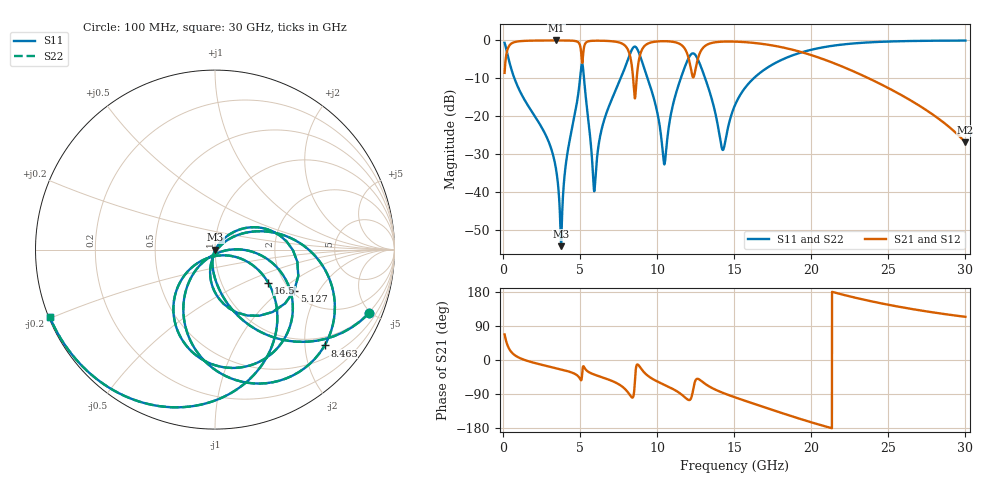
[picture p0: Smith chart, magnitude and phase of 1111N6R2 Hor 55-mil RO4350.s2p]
# GHz S MA R 50
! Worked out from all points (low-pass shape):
!   3201 points, 100 MHz to 30 GHz, reference 50 ohm
!   highest |S21| = -0.02 dB at 3.464 GHz (marker M1); lowest = -26.9 dB at 30 GHz (marker M2)
!   |S21| within 3 dB of the highest: 248.2 MHz to 5.061 GHz (4.813 GHz wide, 181 % of centre); 12.81 GHz to 19.3 GHz (6.488 GHz wide, 40.4 % of centre)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
!   lowest |S11| = -54.3 dB at 3.763 GHz (marker M3), VSWR 1.00, Z = 50.2 - j0.0862 ohm
!   |S11| at or under -10 dB: 733.6 MHz to 4.999 GHz (4.265 GHz wide, 149 % of centre); 5.251 GHz to 7.637 GHz (2.385 GHz wide, 37 % of centre); 13.11 GHz to 16.27 GHz (3.152 GHz wide, 21.5 % of centre)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
!   |S22| runs from -54.3 to 0.0 dB; largest |S21 - S12| = 0
!   S11 on the Smith chart (normalised r, x): 100 MHz: 0.95, -4.84; 5.127 GHz: 2.07, -1.26; 8.463 GHz: 0.78, -2.45; 16.5 GHz: 1.66, -0.69; 30 GHz: 0.00, -0.20
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0.1  0.9278 -22.6  0.3727 67.4  0.3727 67.4  0.9278 -22.6
0.810125  0.2879 -78.6  0.957 11.3  0.957 11.3  0.2879 -78.6
3.46375  0.01843 -107.0  0.9979 -21.8  0.9979 -21.8  0.01843 -107.0
3.76275  0.001918 -26.6  0.9976 -24.8  0.9976 -24.8  0.001918 -26.6
5.089563  0.4641 -8.5  0.6097 -51.8  0.6097 -51.8  0.4641 -8.5
5.126938  0.4971 -27.4  0.5078 -39.4  0.5078 -39.4  0.4971 -27.4
5.939844  0.01075 -15.4  0.9895 -38.8  0.9895 -38.8  0.01075 -15.4
6.500469  0.08074 37.7  0.9881 -46.7  0.9881 -46.7  0.08074 37.7
7.817938  0.391 11.8  0.8846 -73.0  0.8846 -73.0  0.391 11.8
8.462656  0.8115 -41.2  0.2736 -94.6  0.2736 -94.6  0.8115 -41.2
9.041969  0.5071 -106.8  0.7727 -27.4  0.7727 -27.4  0.5071 -106.8
10.06978  0.09632 -133.5  0.9706 -57.9  0.9706 -57.9  0.09632 -133.5
10.49025  0.02372 -53.1  0.9757 -66.0  0.9757 -66.0  0.02372 -53.1
11.54609  0.3225 -12.6  0.8775 -90.0  0.8775 -90.0  0.3225 -12.6
12.29359  0.6734 -70.2  0.3349 -87.0  0.3349 -87.0  0.6734 -70.2
12.86356  0.4359 -121.8  0.741 -55.3  0.741 -55.3  0.4359 -121.8
14.22775  0.03619 -89.8  0.9624 -86.1  0.9624 -86.1  0.03619 -89.8
15.05  0.1399 -19.2  0.963 -98.5  0.963 -98.5  0.1399 -19.2
16.49828  0.3485 -31.8  0.9157 -118.5  0.9157 -118.5  0.3485 -31.8
20.03956  0.7553 -76.2  0.6356 -164.9  0.6356 -164.9  0.7553 -76.2
25.01978  0.9657 -125.4  0.2335 145.6  0.2335 145.6  0.9657 -125.4
30  0.9945 -157.8  0.04497 113.9  0.04497 113.9  0.9945 -157.8
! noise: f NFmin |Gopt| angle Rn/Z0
0.1  0.001077  0.8355  3.108  0.001383
3.417  0.01011  0.4918  22.88  0.003297
6.743  0.03236  0.6604  42.95  0.01588
10.06  0.06499  0.7425  63.46  0.03694
13.39  0.1326  0.8281  81.97  0.09313
16.7  0.07748  0.6721  97.25  0.02086
20.03  0.09525  0.6938  110.9  0.02088
23.35  0.1438  0.7767  125.5  0.02923
26.67  0.2711  0.8758  141.9  0.05213
30  0.813  0.9578  158.7  0.1517
